(* Logix 5000 AddOnInstructionDefinition export HI1734_Faceplate_Standard_AOI; software revision 30.00; part 2 of 2 *)
(* tags used below, declared in another part *)
   Inp_hi1734 : HI:1734_WS:I:0;   // Module Input table
   Out_hi1734 : HI:1734_WS:O:0;   // Module Output table
   rd_az : BOOL;   // Read zero parameters trigger
   pm_6301 : DINT;   // Auto Zero Enable
   pm_6302 : REAL;   // Auto Zero tolerance
   pm_2886 : REAL;   // Zero Tolerance
   pm_6183 : REAL;   // Tare Weight
   rd_inst : BOOL;   // Read Instrument setup parameter trigger
   pm_2881 : DINT;   // Units of measure
   pm_2887 : REAL;   // Motion Tolerance
   save_az_pm : BOOL;   // Save zero parameters trigger
   save_ins_pm : BOOL;   // Save Instrument setup settings trigger
   wr_zero_tolerance_1 : BOOL;   // processs control bit
   wr_tare_weight_1 : BOOL;   // processs control bit
   wr_motion_tolerance_1 : BOOL;   // processs control bit
   wr_units_measure_1 : BOOL;   // processs control bit
   wr_auto_zero_enable_1 : BOOL;   // processs control bit
   wr_auto_zero_tolerance_1 : BOOL;   // processs control bit
   cmd_no : INT;   // Cmd number being sent to module
   check_status_wr_zero_tolerance : BOOL;   // triggers status check of write of parameter
   start_delay_wr_zero_tolerance : BOOL;   // processs control bit
   delay_wr_zero_tolerance : TIMER;   // Delay timer to allow time for process to complete
   check_status_wr_tare_weight : BOOL;   // triggers status check of write of parameter
   start_delay_wr_tare_weight : BOOL;   // processs control bit
   delay_wr_tare_weight : TIMER;   // Delay timer to allow time for process to complete
   check_status_wr_auto_zero_enable : BOOL;   // triggers status check of write parameter
   start_delay_wr_auto_zero_enable : BOOL;   // processs control bit
   delay_wr_auto_zero_enable : TIMER;   // Delay timer to allow time for process to complete
   start_delay_wr_auto_zero_tolerance : BOOL;   // processs control bit
   check_status_wr_auto_zero_tolerance : BOOL;   // triggers status check of write of parameter
   delay_wr_auto_zero_tolerance : TIMER;   // Delay timer to allow time for process to complete
   check_status_wr_motion_tolerance : BOOL;   // triggers status check of write of parameter
   start_delay_wr_motion_toleranc : BOOL;   // processs control bit
   delay_wr_motion_toleranc : TIMER;   // Delay timer to allow time for process to complete
   check_status_wr_units_measure : BOOL;   // triggers status check of write of parameter
   start_delay_wr_units_measure : BOOL;   // processs control bit
   delay_wr_units_measure : TIMER;   // Delay timer to allow time for process to complete
   wr_auto_zero_enable_2 : BOOL;   // processs control bit
   wr_auto_zero_tolerance_2 : BOOL;   // processs control bit
   wr_zero_tolerance_2 : BOOL;   // processs control bit
   wr_units_measure_2 : BOOL;   // processs control bit
   wr_motion_tolerance_2 : BOOL;   // processs control bit
   wr_tare_weight_2 : BOOL;   // processs control bit
   ons_15 : BOOL;   // processs control bit
(* HI1734_Faceplate_Standard_AOI, continued *)

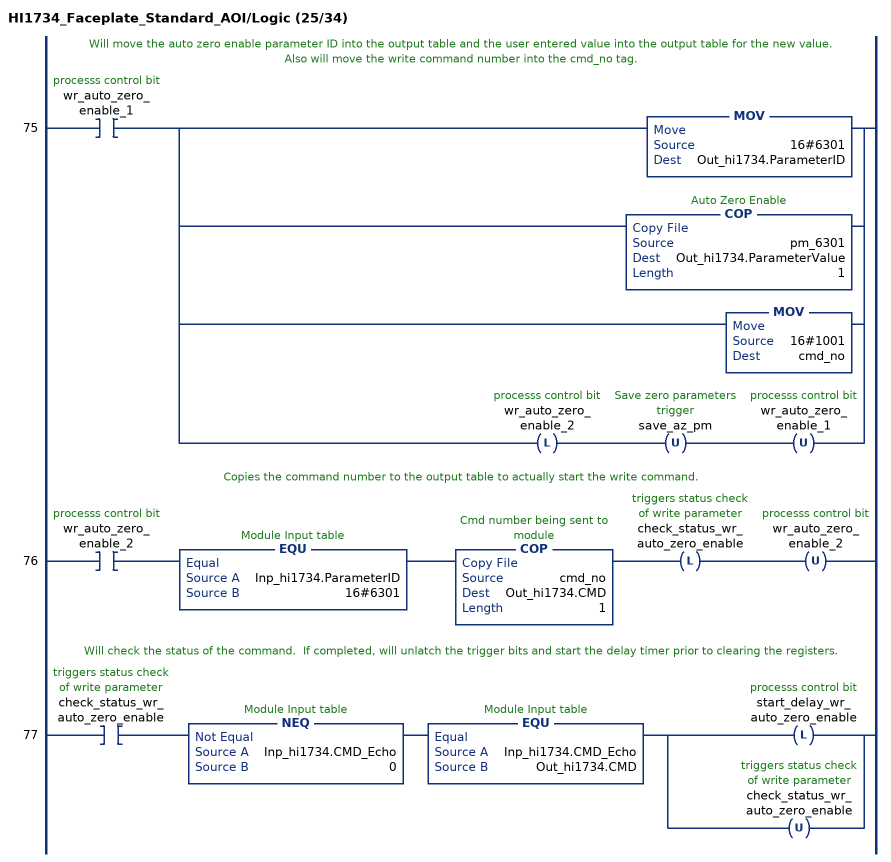
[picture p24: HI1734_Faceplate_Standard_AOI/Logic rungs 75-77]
   // Will move the auto zero enable parameter ID into the output table and the user entered value into the output table for the new value.  Also will move the write command number into the cmd_no tag.
   75: XIC(wr_auto_zero_enable_1)[MOV(16#6301,Out_hi1734.ParameterID) ,COP(pm_6301,Out_hi1734.ParameterValue,1) ,MOV(16#1001,cmd_no) ,OTL(wr_auto_zero_enable_2) OTU(save_az_pm) OTU(wr_auto_zero_enable_1) ];
   // Copies the command number to the output table to actually start the write command.
   76: XIC(wr_auto_zero_enable_2)EQU(Inp_hi1734.ParameterID,16#6301)COP(cmd_no,Out_hi1734.CMD,1)OTL(check_status_wr_auto_zero_enable)OTU(wr_auto_zero_enable_2);
   // Will check the status of the command.  If completed, will unlatch the trigger bits and start the delay timer prior to clearing the registers.
   77: XIC(check_status_wr_auto_zero_enable)NEQ(Inp_hi1734.CMD_Echo,0)EQU(Inp_hi1734.CMD_Echo,Out_hi1734.CMD)[OTL(start_delay_wr_auto_zero_enable) ,OTU(check_status_wr_auto_zero_enable) ];
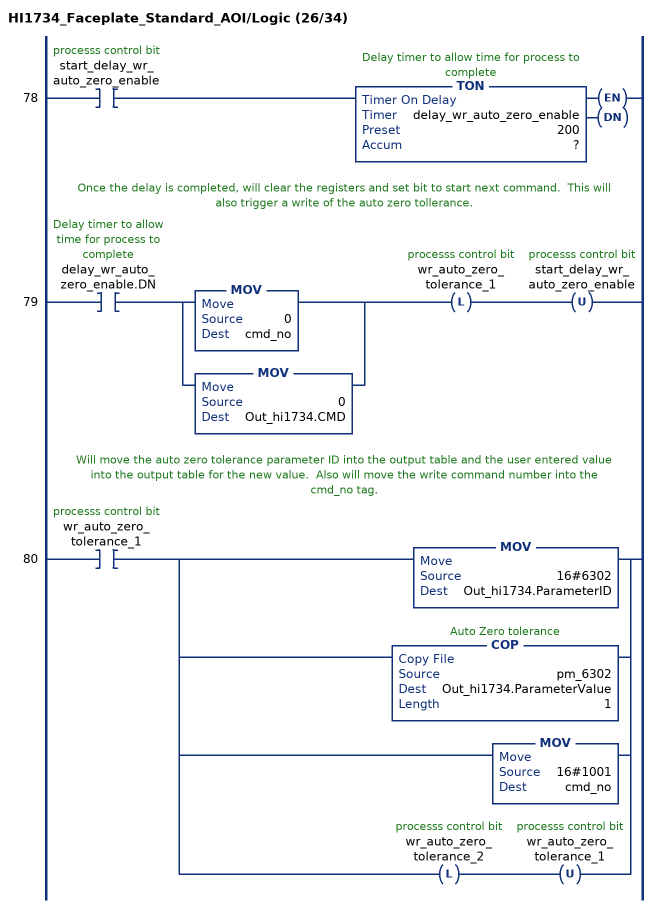
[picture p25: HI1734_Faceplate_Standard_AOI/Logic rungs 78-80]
   78: XIC(start_delay_wr_auto_zero_enable)TON(delay_wr_auto_zero_enable,?,?);
   // Once the delay is completed, will clear the registers and set bit to start next command.  This will also trigger a write of the auto zero tollerance.
   79: XIC(delay_wr_auto_zero_enable.DN)[MOV(0,cmd_no) ,MOV(0,Out_hi1734.CMD) ]OTL(wr_auto_zero_tolerance_1)OTU(start_delay_wr_auto_zero_enable);
   // Will move the auto zero tolerance parameter ID into the output table and the user entered value into the output table for the new value.  Also will move the write command number into the cmd_no tag.
   80: XIC(wr_auto_zero_tolerance_1)[MOV(16#6302,Out_hi1734.ParameterID) ,COP(pm_6302,Out_hi1734.ParameterValue,1) ,MOV(16#1001,cmd_no) ,OTL(wr_auto_zero_tolerance_2) OTU(wr_auto_zero_tolerance_1) ];
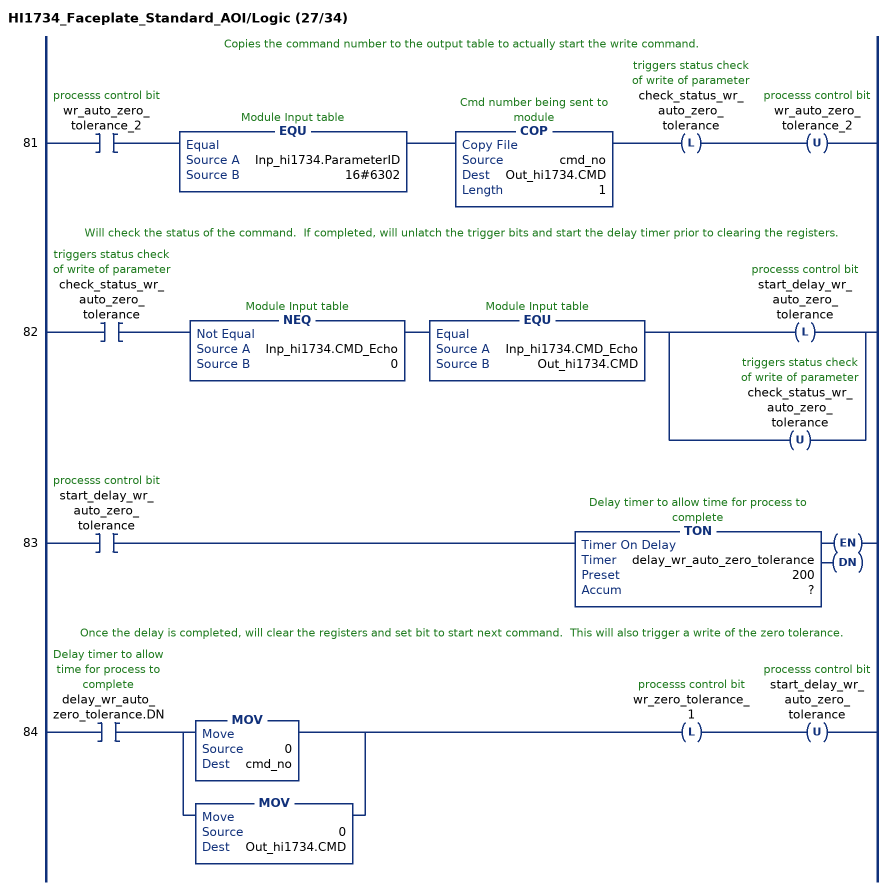
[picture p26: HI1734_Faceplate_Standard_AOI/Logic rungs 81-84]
   // Copies the command number to the output table to actually start the write command.
   81: XIC(wr_auto_zero_tolerance_2)EQU(Inp_hi1734.ParameterID,16#6302)COP(cmd_no,Out_hi1734.CMD,1)OTL(check_status_wr_auto_zero_tolerance)OTU(wr_auto_zero_tolerance_2);
   // Will check the status of the command.  If completed, will unlatch the trigger bits and start the delay timer prior to clearing the registers.
   82: XIC(check_status_wr_auto_zero_tolerance)NEQ(Inp_hi1734.CMD_Echo,0)EQU(Inp_hi1734.CMD_Echo,Out_hi1734.CMD)[OTL(start_delay_wr_auto_zero_tolerance) ,OTU(check_status_wr_auto_zero_tolerance) ];
   83: XIC(start_delay_wr_auto_zero_tolerance)TON(delay_wr_auto_zero_tolerance,?,?);
   // Once the delay is completed, will clear the registers and set bit to start next command.  This will also trigger a write of the zero tolerance.
   84: XIC(delay_wr_auto_zero_tolerance.DN)[MOV(0,cmd_no) ,MOV(0,Out_hi1734.CMD) ]OTL(wr_zero_tolerance_1)OTU(start_delay_wr_auto_zero_tolerance);
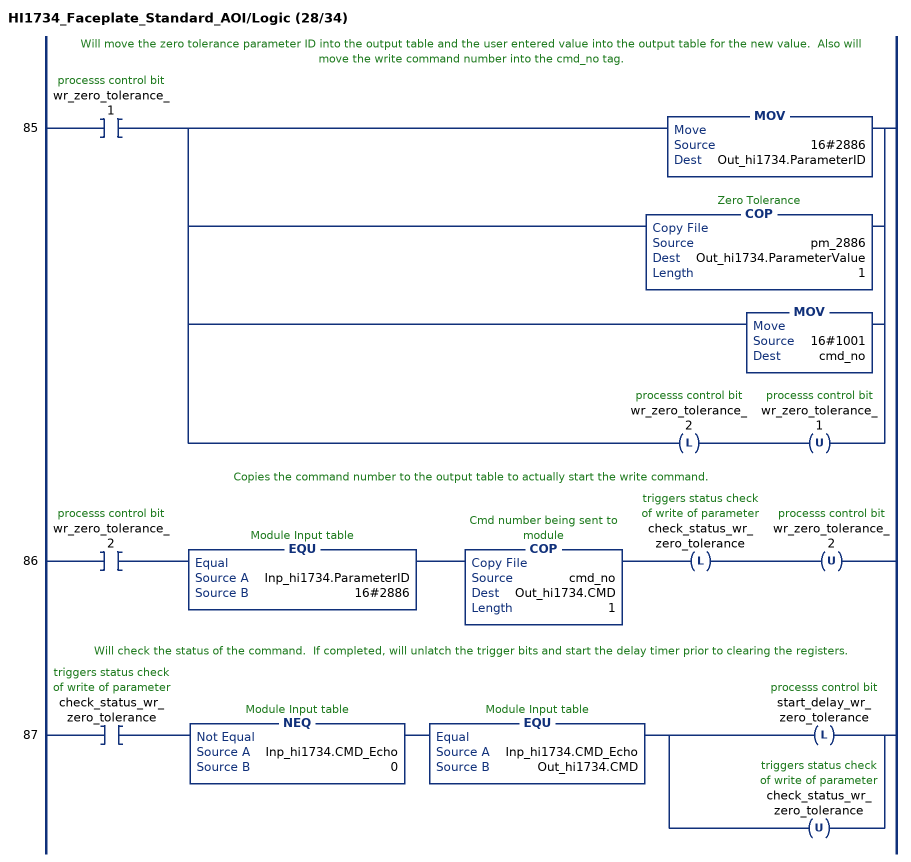
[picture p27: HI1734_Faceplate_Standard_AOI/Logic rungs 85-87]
   // Will move the zero tolerance parameter ID into the output table and the user entered value into the output table for the new value.  Also will move the write command number into the cmd_no tag.
   85: XIC(wr_zero_tolerance_1)[MOV(16#2886,Out_hi1734.ParameterID) ,COP(pm_2886,Out_hi1734.ParameterValue,1) ,MOV(16#1001,cmd_no) ,OTL(wr_zero_tolerance_2) OTU(wr_zero_tolerance_1) ];
   // Copies the command number to the output table to actually start the write command.
   86: XIC(wr_zero_tolerance_2)EQU(Inp_hi1734.ParameterID,16#2886)COP(cmd_no,Out_hi1734.CMD,1)OTL(check_status_wr_zero_tolerance)OTU(wr_zero_tolerance_2);
   // Will check the status of the command.  If completed, will unlatch the trigger bits and start the delay timer prior to clearing the registers.
   87: XIC(check_status_wr_zero_tolerance)NEQ(Inp_hi1734.CMD_Echo,0)EQU(Inp_hi1734.CMD_Echo,Out_hi1734.CMD)[OTL(start_delay_wr_zero_tolerance) ,OTU(check_status_wr_zero_tolerance) ];
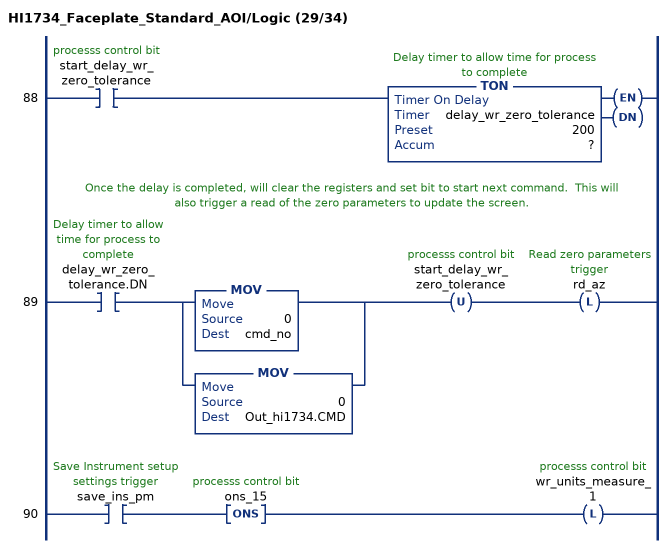
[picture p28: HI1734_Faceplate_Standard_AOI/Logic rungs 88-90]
   88: XIC(start_delay_wr_zero_tolerance)TON(delay_wr_zero_tolerance,?,?);
   // Once the delay is completed, will clear the registers and set bit to start next command.  This will also trigger a read of the zero parameters to update the screen.
   89: XIC(delay_wr_zero_tolerance.DN)[MOV(0,cmd_no) ,MOV(0,Out_hi1734.CMD) ]OTU(start_delay_wr_zero_tolerance)OTL(rd_az);
   90: XIC(save_ins_pm)ONS(ons_15)OTL(wr_units_measure_1);
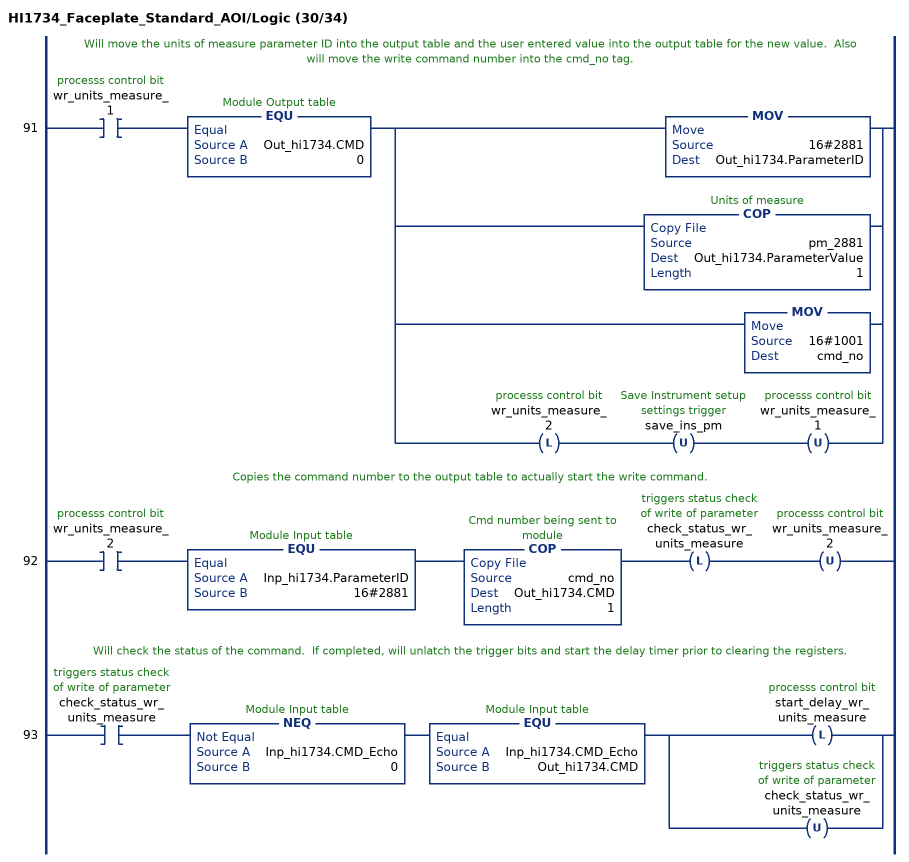
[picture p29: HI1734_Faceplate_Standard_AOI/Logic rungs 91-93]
   // Will move the units of measure parameter ID into the output table and the user entered value into the output table for the new value.  Also will move the write command number into the cmd_no tag.
   91: XIC(wr_units_measure_1)EQU(Out_hi1734.CMD,0)[MOV(16#2881,Out_hi1734.ParameterID) ,COP(pm_2881,Out_hi1734.ParameterValue,1) ,MOV(16#1001,cmd_no) ,OTL(wr_units_measure_2) OTU(save_ins_pm) OTU(wr_units_measure_1) ];
   // Copies the command number to the output table to actually start the write command.
   92: XIC(wr_units_measure_2)EQU(Inp_hi1734.ParameterID,16#2881)COP(cmd_no,Out_hi1734.CMD,1)OTL(check_status_wr_units_measure)OTU(wr_units_measure_2);
   // Will check the status of the command.  If completed, will unlatch the trigger bits and start the delay timer prior to clearing the registers.
   93: XIC(check_status_wr_units_measure)NEQ(Inp_hi1734.CMD_Echo,0)EQU(Inp_hi1734.CMD_Echo,Out_hi1734.CMD)[OTL(start_delay_wr_units_measure) ,OTU(check_status_wr_units_measure) ];
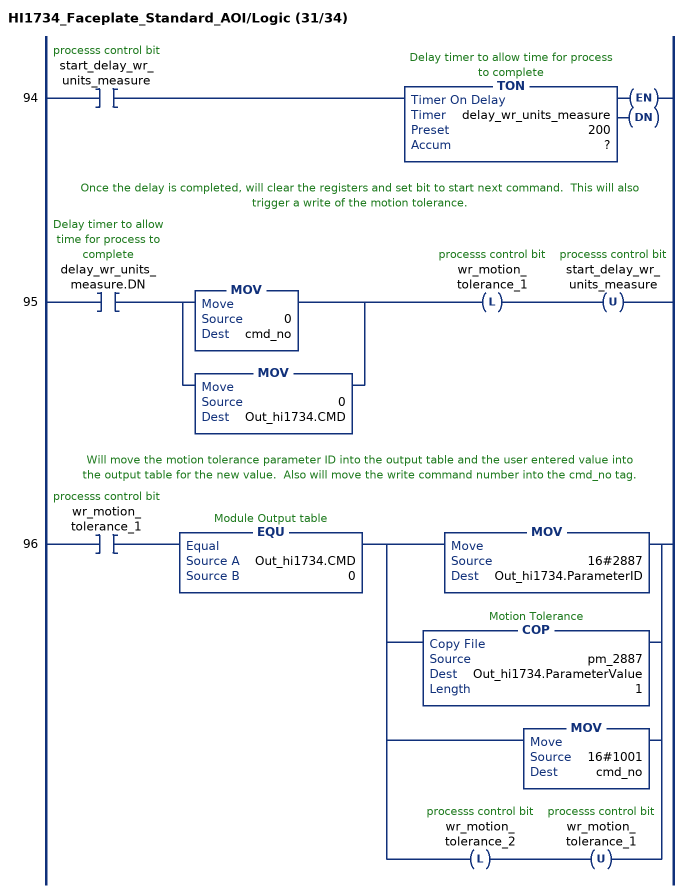
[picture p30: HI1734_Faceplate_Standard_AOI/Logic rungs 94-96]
   94: XIC(start_delay_wr_units_measure)TON(delay_wr_units_measure,?,?);
   // Once the delay is completed, will clear the registers and set bit to start next command.  This will also trigger a write of the motion tolerance.
   95: XIC(delay_wr_units_measure.DN)[MOV(0,cmd_no) ,MOV(0,Out_hi1734.CMD) ]OTL(wr_motion_tolerance_1)OTU(start_delay_wr_units_measure);
   // Will move the motion tolerance parameter ID into the output table and the user entered value into the output table for the new value.  Also will move the write command number into the cmd_no tag.
   96: XIC(wr_motion_tolerance_1)EQU(Out_hi1734.CMD,0)[MOV(16#2887,Out_hi1734.ParameterID) ,COP(pm_2887,Out_hi1734.ParameterValue,1) ,MOV(16#1001,cmd_no) ,OTL(wr_motion_tolerance_2) OTU(wr_motion_tolerance_1) ];
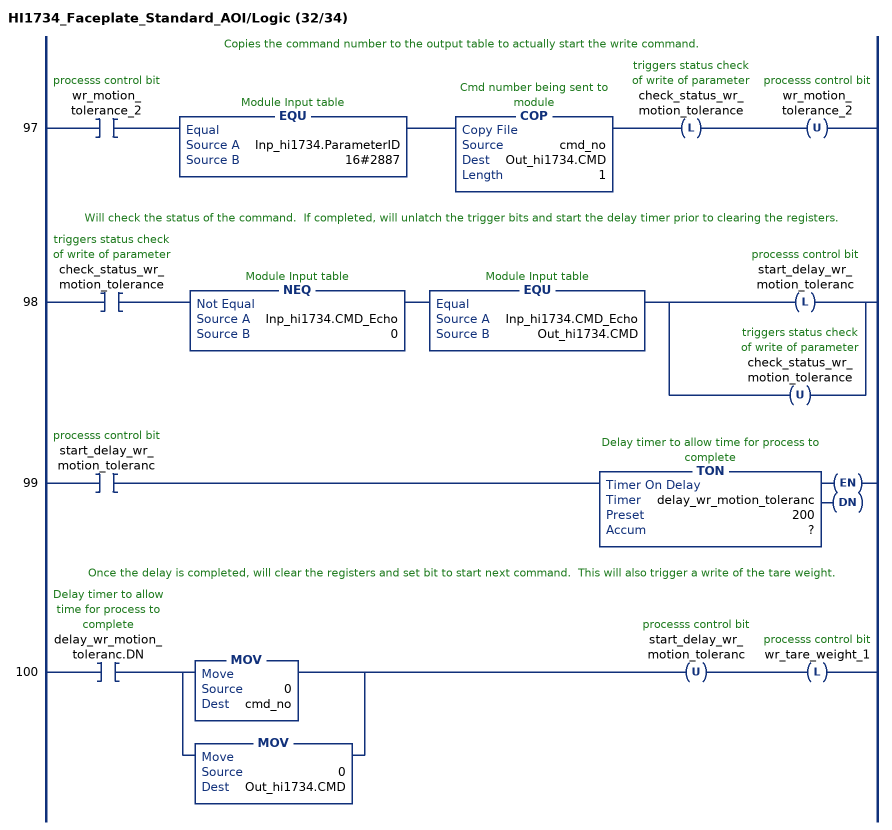
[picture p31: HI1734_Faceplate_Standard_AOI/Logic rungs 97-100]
   // Copies the command number to the output table to actually start the write command.
   97: XIC(wr_motion_tolerance_2)EQU(Inp_hi1734.ParameterID,16#2887)COP(cmd_no,Out_hi1734.CMD,1)OTL(check_status_wr_motion_tolerance)OTU(wr_motion_tolerance_2);
   // Will check the status of the command.  If completed, will unlatch the trigger bits and start the delay timer prior to clearing the registers.
   98: XIC(check_status_wr_motion_tolerance)NEQ(Inp_hi1734.CMD_Echo,0)EQU(Inp_hi1734.CMD_Echo,Out_hi1734.CMD)[OTL(start_delay_wr_motion_toleranc) ,OTU(check_status_wr_motion_tolerance) ];
   99: XIC(start_delay_wr_motion_toleranc)TON(delay_wr_motion_toleranc,?,?);
   // Once the delay is completed, will clear the registers and set bit to start next command.  This will also trigger a write of the tare weight.
   100: XIC(delay_wr_motion_toleranc.DN)[MOV(0,cmd_no) ,MOV(0,Out_hi1734.CMD) ]OTU(start_delay_wr_motion_toleranc)OTL(wr_tare_weight_1);
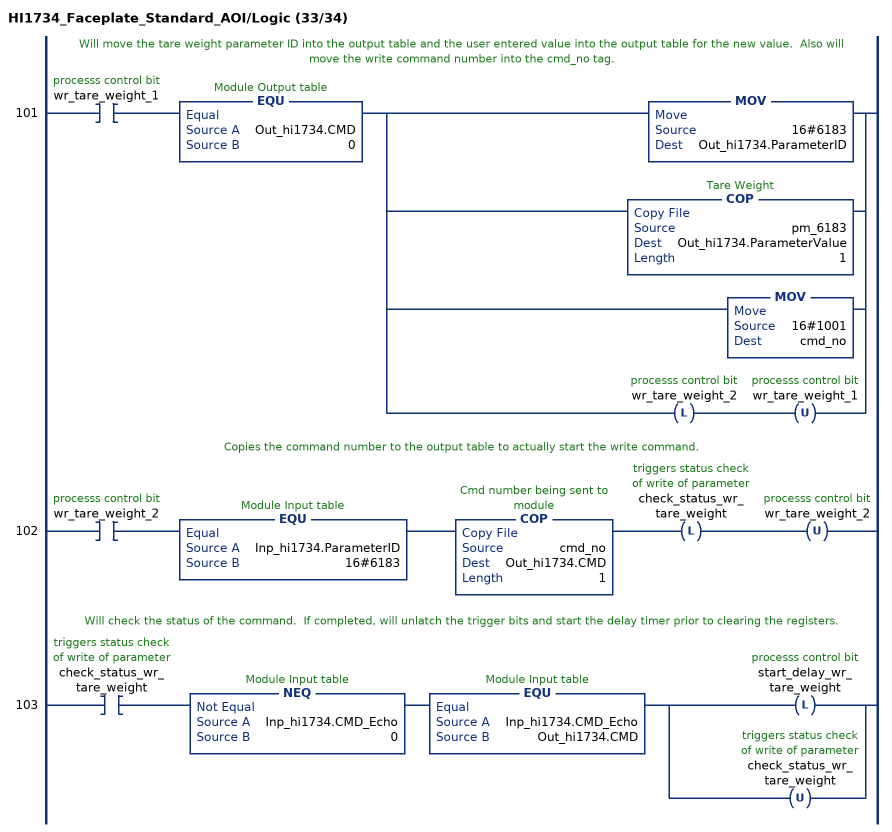
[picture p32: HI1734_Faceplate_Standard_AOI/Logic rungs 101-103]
   // Will move the tare weight parameter ID into the output table and the user entered value into the output table for the new value.  Also will move the write command number into the cmd_no tag.
   101: XIC(wr_tare_weight_1)EQU(Out_hi1734.CMD,0)[MOV(16#6183,Out_hi1734.ParameterID) ,COP(pm_6183,Out_hi1734.ParameterValue,1) ,MOV(16#1001,cmd_no) ,OTL(wr_tare_weight_2) OTU(wr_tare_weight_1) ];
   // Copies the command number to the output table to actually start the write command.
   102: XIC(wr_tare_weight_2)EQU(Inp_hi1734.ParameterID,16#6183)COP(cmd_no,Out_hi1734.CMD,1)OTL(check_status_wr_tare_weight)OTU(wr_tare_weight_2);
   // Will check the status of the command.  If completed, will unlatch the trigger bits and start the delay timer prior to clearing the registers.
   103: XIC(check_status_wr_tare_weight)NEQ(Inp_hi1734.CMD_Echo,0)EQU(Inp_hi1734.CMD_Echo,Out_hi1734.CMD)[OTL(start_delay_wr_tare_weight) ,OTU(check_status_wr_tare_weight) ];
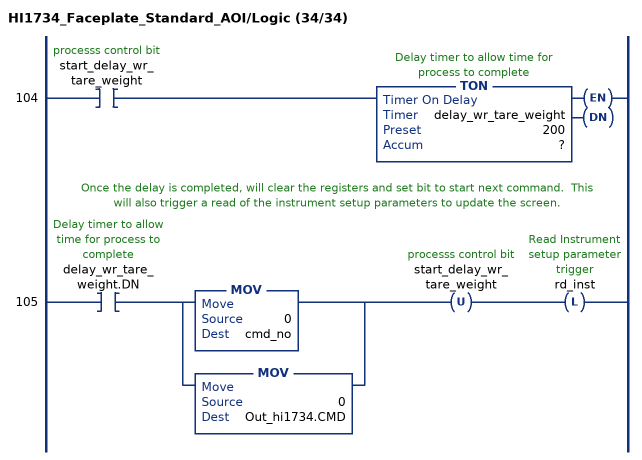
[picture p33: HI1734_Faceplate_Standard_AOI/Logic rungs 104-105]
   104: XIC(start_delay_wr_tare_weight)TON(delay_wr_tare_weight,?,?);
   // Once the delay is completed, will clear the registers and set bit to start next command.  This will also trigger a read of the instrument setup parameters to update the screen.
   105: XIC(delay_wr_tare_weight.DN)[MOV(0,cmd_no) ,MOV(0,Out_hi1734.CMD) ]OTU(start_delay_wr_tare_weight)OTL(rd_inst);
END_ROUTINE
END_ADD_ON_INSTRUCTION
